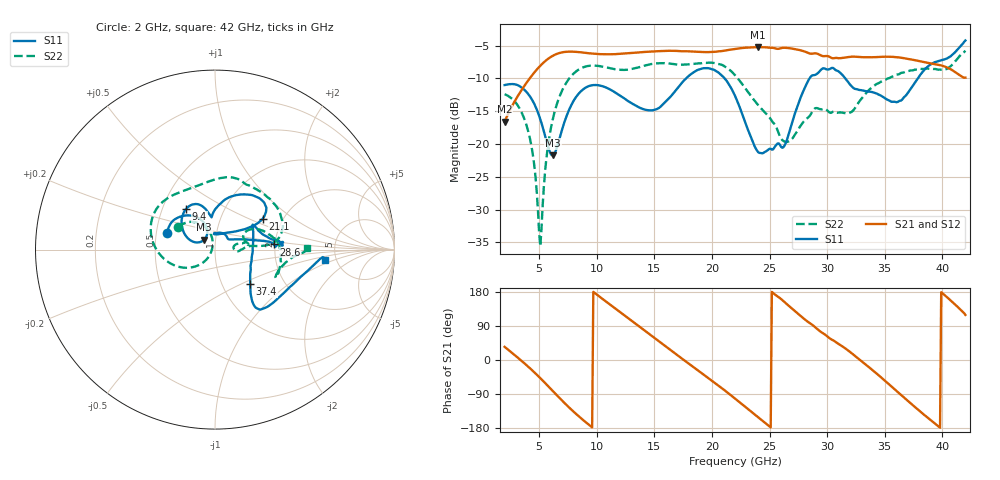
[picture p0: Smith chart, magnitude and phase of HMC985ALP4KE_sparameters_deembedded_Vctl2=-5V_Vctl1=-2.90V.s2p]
!s2p File: Measurements: S11, S21, S12, S22
# GHz S dB R 50.0
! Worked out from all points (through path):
!   401 points, 2 GHz to 42 GHz, reference 50 ohm
!   highest |S21| = -5.22 dB at 24 GHz (marker M1); lowest = -16.6 dB at 2 GHz (marker M2)
!   lowest |S11| = -21.7 dB at 6.2 GHz (marker M3), VSWR 1.18, Z = 44 + j4.84 ohm
!   |S11| at or under -10 dB: start of sweep to 17.75 GHz; 21.11 GHz to 28.47 GHz (7.36 GHz wide, 29.7 % of centre); 31.58 GHz to 37.86 GHz (6.287 GHz wide, 18.1 % of centre)
!   |S22| runs from -35.6 to -5.8 dB; largest |S21 - S12| = 0.00066
!   S11 on the Smith chart (normalised r, x): 2 GHz: 0.57, +0.12; 9.4 GHz: 0.66, +0.32; 21.1 GHz: 1.58, +0.61; 28.6 GHz: 1.97, +0.13; 37.4 GHz: 1.35, -0.57; 42 GHz: 4.08, -0.73
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2  -11.00 160.5  -16.61 34.7  -16.61 34.7  -12.40 148.7
4  -12.26 128.5  -10.41 -16.3  -10.41 -16.3  -17.73 111.9
5.1  -16.22 111.8  -8.05 -47.9  -8.05 -47.9  -35.57 171.0
5.7  -19.96 115.4  -7.10 -66.5  -7.10 -66.5  -21.14 -131.6
6.2  -21.72 138.2  -6.52 -82.3  -6.52 -82.3  -16.07 -141.7
8.7  -11.83 135.8  -6.03 -155.4  -6.03 -155.4  -8.38 160.0
9.4  -11.11 125.4  -6.17 -172.9  -6.17 -172.9  -8.05 148.3
12.7  -13.43 100.9  -6.17 111.1  -6.17 111.1  -8.66 104.6
15.4  -14.49 95.1  -5.84 49.2  -5.84 49.2  -7.67 75.7
18  -9.59 67.1  -5.86 -9.9  -5.87 -9.9  -7.83 58.5
21.1  -9.99 32.9  -5.75 -80.0  -5.75 -79.9  -8.16 16.5
22  -12.63 32.6  -5.49 -101.7  -5.50 -101.7  -9.49 7.4
24  -21.21 78.3  -5.22 -150.6  -5.22 -150.6  -14.03 5.8
26.4  -19.88 33.7  -5.32 150.1  -5.32 150.1  -19.67 4.4
28.6  -9.67 5.0  -6.22 95.1  -6.23 95.1  -15.40 13.5
28.7  -9.53 3.7  -6.21 93.0  -6.22 93.1  -15.06 13.4
30.5  -8.38 5.9  -6.92 52.2  -6.92 52.2  -15.07 15.1
32.4  -11.57 23.7  -6.67 11.1  -6.67 11.1  -14.55 29.4
35.4  -13.37 8.7  -6.68 -64.9  -6.68 -64.9  -9.92 14.3
37.4  -11.20 -44.6  -7.14 -118.4  -7.14 -118.3  -8.77 -2.2
39.7  -7.31 -48.1  -7.92 -176.2  -7.92 -176.1  -8.65 -24.5
42  -4.20 -5.2  -9.87 119.0  -9.87 119.0  -5.77 1.3
